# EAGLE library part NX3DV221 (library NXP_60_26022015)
High-speed USB 2.0 switch with enable
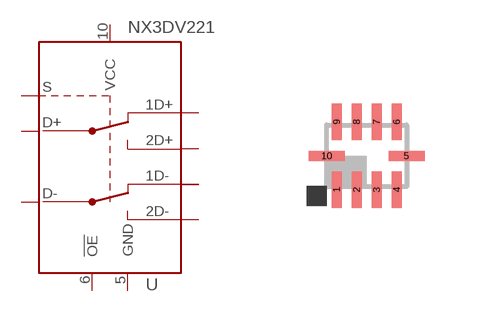
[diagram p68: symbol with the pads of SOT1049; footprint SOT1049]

Designator prefix U

## NX3DV221GM  [SOT1049]
1  1D+  out
2  1D-  out
3  2D+  out
4  2D-  out
5  GND  out
6  !OE!  out
7  D-  out
8  D+  out
9  S  out
10  VCC  out

## Footprint SOT1049 (pad centres in mm)
SOT1049 XQFN10U: plastic extremely thin quad flat package; no leads; 10 terminals; UTLP based; body 2 x 1.55 x 0.5 mm JEDEC: MO-255 IEC: --
smd 0.25 x 0.9: 1 -0.75,-0.85; 2 -0.25,-0.85; 3 0.25,-0.85; 4 0.75,-0.85; 6 0.75,0.85; 7 0.25,0.85; 8 -0.25,0.85; 9 -0.75,0.85
smd 0.9 x 0.25: 5 1,0; 10 -1,0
